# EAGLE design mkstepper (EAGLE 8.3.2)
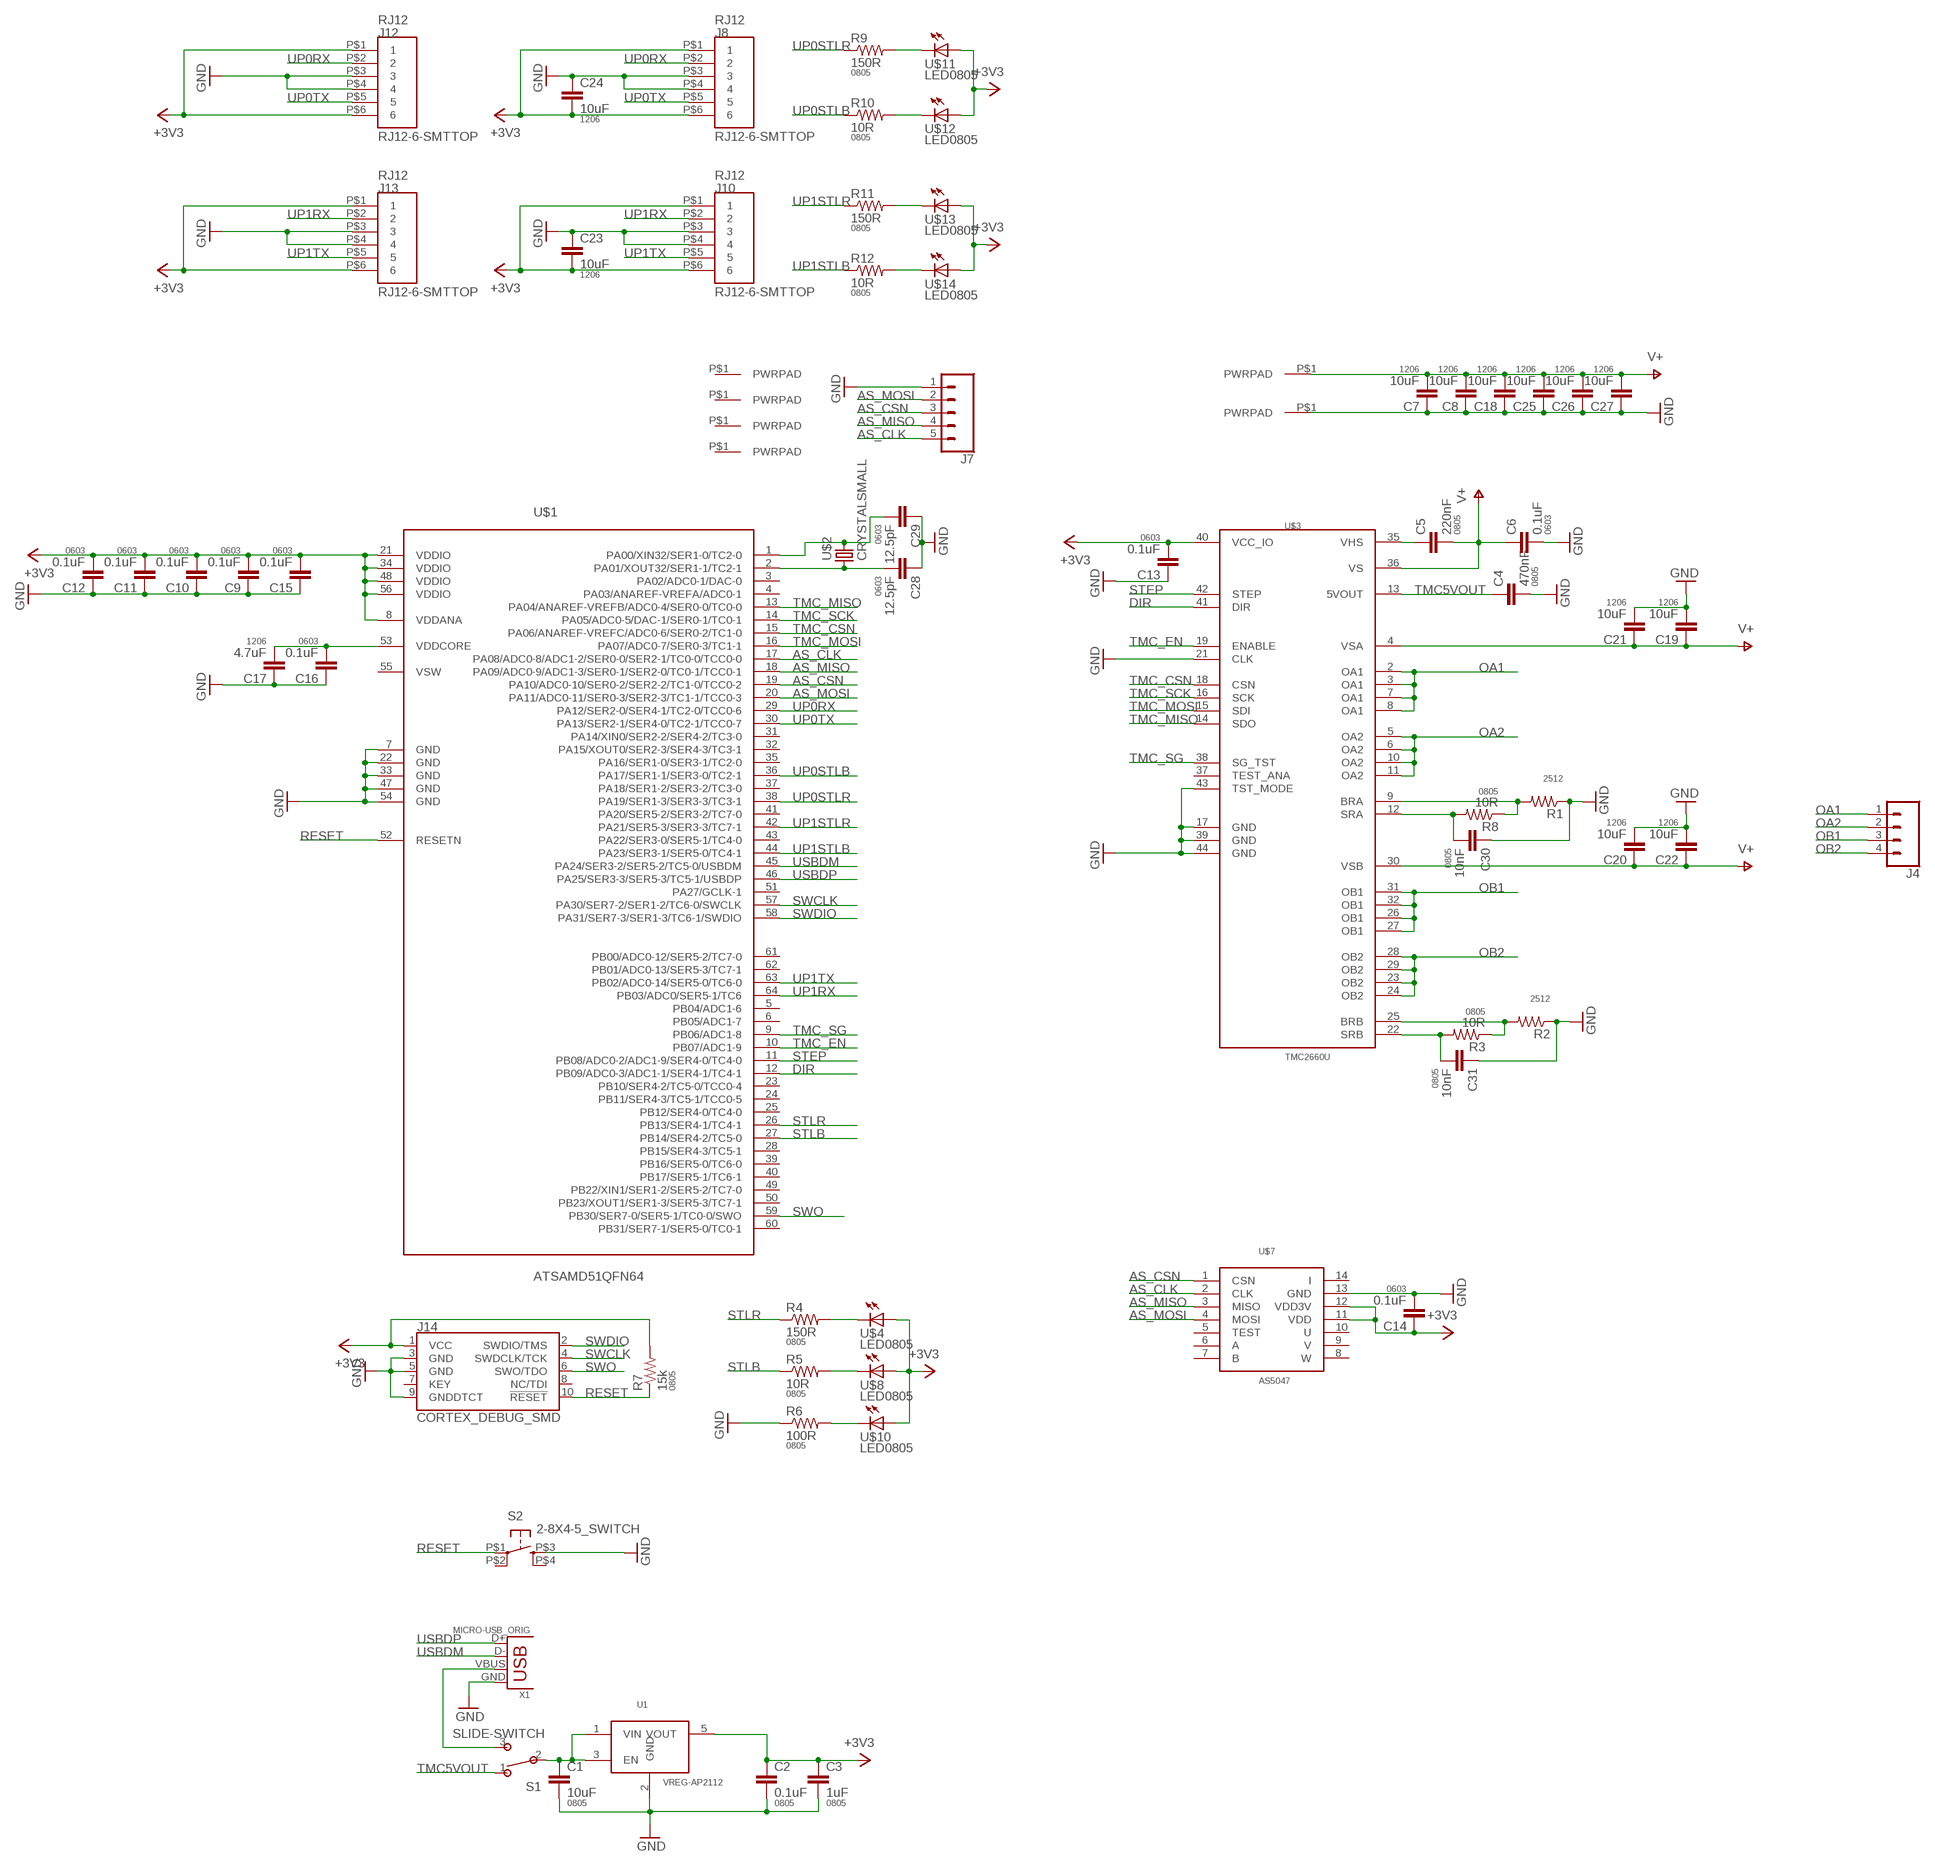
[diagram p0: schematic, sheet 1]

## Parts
C1  10uF  CAP0805  [0805]
C2  0.1uF  CAP0805  [0805]
C3  1uF  CAP0805  [0805]
C4  470nF  CAP0805  [0805]
C5  220nF  CAP0805  [0805]
C6  0.1uF  CAP0603-CAP  [0603-CAP]
C7  10uF  CAP1206  [1206]
C8  10uF  CAP1206  [1206]
C9  0.1uF  CAP0603-CAP  [0603-CAP]
C10  0.1uF  CAP0603-CAP  [0603-CAP]
C11  0.1uF  CAP0603-CAP  [0603-CAP]
C12  0.1uF  CAP0603-CAP  [0603-CAP]
C13  0.1uF  CAP0603-CAP  [0603-CAP]
C14  0.1uF  CAP0603-CAP  [0603-CAP]
C15  0.1uF  CAP0603-CAP  [0603-CAP]
C16  0.1uF  CAP0603-CAP  [0603-CAP]
C17  4.7uF  CAP1206  [1206]
C18  10uF  CAP1206  [1206]
C19  10uF  CAP1206  [1206]
C20  10uF  CAP1206  [1206]
C21  10uF  CAP1206  [1206]
C22  10uF  CAP1206  [1206]
C23  10uF  CAP1206  [1206]
C24  10uF  CAP1206  [1206]
C25  10uF  CAP1206  [1206]
C26  10uF  CAP1206  [1206]
C27  10uF  CAP1206  [1206]
C28  12.5pF  CAP0603-CAP  [0603-CAP]
C29  12.5pF  CAP0603-CAP  [0603-CAP]
C30  10nF  CAP0805  [0805]
C31  10nF  CAP0805  [0805]
J2  PWRPAD  [PWRPAD_M3-PEM-MOUNT]
J3  PWRPAD  [PWRPAD_M3-PEM-MOUNT]
J4  CONN_04LONGPADS  [1X04_LONGPADS]
J5  PWRPADM3  [PWRPAD_3-25MM]
J6  PWRPADM3  [PWRPAD_3-25MM]
J7  CONN_05NO_SILK  [1X05_NO_SILK]
J8  RJ12-6-SMTTOP  [RJ12-6-SMT-TOPENTRY]
J9  PWRPADM3  [PWRPAD_3-25MM]
J10  RJ12-6-SMTTOP  [RJ12-6-SMT-TOPENTRY]
J11  PWRPADM3  [PWRPAD_3-25MM]
J12  RJ12-6-SMTTOP  [RJ12-6-SMT-TOPENTRY]
J13  RJ12-6-SMTTOP  [RJ12-6-SMT-TOPENTRY]
J14  CORTEX_DEBUG_SMD  [SAMTECH_FTSH-105-01]
R1  RESISTOR2512  [R2512]
R2  RESISTOR2512  [R2512]
R3  10R  RESISTOR0805-RES  [0805]
R4  150R  RESISTOR0805-RES  [0805]
R5  10R  RESISTOR0805-RES  [0805]
R6  100R  RESISTOR0805-RES  [0805]
R7  15k  RESISTOR0805-RES  [0805]
R8  10R  RESISTOR0805-RES  [0805]
R9  150R  RESISTOR0805-RES  [0805]
R10  10R  RESISTOR0805-RES  [0805]
R11  150R  RESISTOR0805-RES  [0805]
R12  10R  RESISTOR0805-RES  [0805]
S1  SLIDE-SWITCH  [AYZ0102AGRLC]
S2  2-8X4-5_SWITCH  [TACT-SWITCH-KMR6]
U1  VREG-AP2112  [SOT23-5]
U$1  ATSAMD51QFN64  [QFN-64-9X9MM]
U$2  CRYSTALSMALL  [2-SMD-1-5X3-2MM]
U$3  TMC2660U  [TQFP44]
U$4  LED0805  [LED0805]
U$7  AS5047  [TSSOP14]
U$8  LED0805  [LED0805]
U$10  LED0805  [LED0805]
U$11  LED0805  [LED0805]
U$12  LED0805  [LED0805]
U$13  LED0805  [LED0805]
U$14  LED0805  [LED0805]
X1  MICRO-USB_ORIG  [DX4R005HJ5]

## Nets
+3V3: C2.1 C3.1 C9.2 C10.2 C11.2 C12.2 C13.2 C14.1 C15.2 C23.2 C24.2 J8.P$1 J8.P$6 J10.P$1 J10.P$6 J12.P$1 J12.P$6 J13.P$1 J13.P$6 J14.1(VCC) R7.2 U1.5(VOUT) U$1.8(VDDANA) U$1.21(VDDIO) U$1.34(VDDIO) U$1.48(VDDIO) U$1.56(VDDIO) U$3.40(VCC_IO) U$4.1(A) U$7.11(VDD) U$7.12(VDD3V) U$8.1(A) U$10.1(A) U$11.1(A) U$12.1(A) U$13.1(A) U$14.1(A)
AS_CLK: J7.5 U$1.17(PA08/ADC0-8/ADC1-2/SER0-0/SER2-1/TC0-0/TCC0-0) U$7.2(CLK)
AS_CSN: J7.3 U$1.19(PA10/ADC0-10/SER0-2/SER2-2/TC1-0/TCC0-2) U$7.1(CSN)
AS_MISO: J7.4 U$1.18(PA09/ADC0-9/ADC1-3/SER0-1/SER2-0/TC0-1/TCC0-1) U$7.3(MISO)
AS_MOSI: J7.2 U$1.20(PA11/ADC0-11/SER0-3/SER2-3/TC1-1/TCC0-3) U$7.4(MOSI)
BRA: R1.2 R8.1 U$3.9(BRA)
BRB: R2.2 R3.1 U$3.25(BRB)
DIR: U$1.12(PB09/ADC0-3/ADC1-1/SER4-1/TC4-1) U$3.41(DIR)
GND: C1.2 C2.2 C3.2 C4.2 C6.2 C7.1 C8.1 C9.1 C10.1 C11.1 C12.1 C13.1 C14.2 C15.1 C16.1 C17.1 C18.1 C19.2 C20.2 C21.2 C22.2 C23.1 C24.1 C25.1 C26.1 C27.1 C28.1 C29.1 C30.1 C31.1 J3.P$1(PWRPAD) J7.1 J8.P$3 J8.P$4 J10.P$3 J10.P$4 J12.P$3 J12.P$4 J13.P$3 J13.P$4 J14.3(GND) J14.5(GND) J14.9(GNDDTCT) R1.1 R2.1 R6.1 S2.P$3(S) U1.2(GND) U$1.7(GND) U$1.22(GND) U$1.33(GND) U$1.47(GND) U$1.54(GND) U$3.17(GND) U$3.21(CLK) U$3.39(GND) U$3.43(TST_MODE) U$3.44(GND) U$7.13(GND) X1.GND
N$1: R6.2 U$10.2(C)
N$2: C5.1 U$3.35(VHS)
N$3: C1.1 S1.2 U1.1(VIN) U1.3(EN)
N$4: S1.3 X1.VBUS
N$5: R5.2 U$8.2(C)
N$6: R4.2 U$4.2(C)
N$7: C16.2 C17.2 U$1.53(VDDCORE)
N$8: C28.2 U$1.2(PA01/XOUT32/SER1-1/TC2-1) U$2.P$1
N$10: R9.2 U$11.2(C)
N$11: R10.2 U$12.2(C)
N$12: C29.2 U$1.1(PA00/XIN32/SER1-0/TC2-0) U$2.P$2
N$13: R11.2 U$13.2(C)
N$14: R12.2 U$14.2(C)
OA1: J4.1 U$3.2(OA1) U$3.3(OA1) U$3.7(OA1) U$3.8(OA1)
OA2: J4.2 U$3.5(OA2) U$3.6(OA2) U$3.10(OA2) U$3.11(OA2)
OB1: J4.3 U$3.26(OB1) U$3.27(OB1) U$3.31(OB1) U$3.32(OB1)
OB2: J4.4 U$3.23(OB2) U$3.24(OB2) U$3.28(OB2) U$3.29(OB2)
RESET: J14.10(!RESET) R7.1 S2.P$1(P) U$1.52(RESETN)
SRA: C30.2 R8.2 U$3.12(SRA)
SRB: C31.2 R3.2 U$3.22(SRB)
STEP: U$1.11(PB08/ADC0-2/ADC1-9/SER4-0/TC4-0) U$3.42(STEP)
STLB: R5.1 U$1.27(PB14/SER4-2/TC5-0)
STLR: R4.1 U$1.26(PB13/SER4-1/TC4-1)
SWCLK: J14.4(SWDCLK/TCK) U$1.57(PA30/SER7-2/SER1-2/TC6-0/SWCLK)
SWDIO: J14.2(SWDIO/TMS) U$1.58(PA31/SER7-3/SER1-3/TC6-1/SWDIO)
SWO: J14.6(SWO/TDO) U$1.59(PB30/SER7-0/SER5-1/TC0-0/SWO)
TMC5VOUT: C4.1 S1.1 U$3.13(5VOUT)
TMC_CSN: U$1.15(PA06/ANAREF-VREFC/ADC0-6/SER0-2/TC1-0) U$3.18(CSN)
TMC_EN: U$1.10(PB07/ADC1-9) U$3.19(ENABLE)
TMC_MISO: U$1.13(PA04/ANAREF-VREFB/ADC0-4/SER0-0/TC0-0) U$3.14(SDO)
TMC_MOSI: U$1.16(PA07/ADC0-7/SER0-3/TC1-1) U$3.15(SDI)
TMC_SCK: U$1.14(PA05/ADC0-5/DAC-1/SER0-1/TC0-1) U$3.16(SCK)
TMC_SG: U$1.9(PB06/ADC1-8) U$3.38(SG_TST)
UP0RX: J8.P$2 J12.P$2 U$1.29(PA12/SER2-0/SER4-1/TC2-0/TCC0-6)
UP0STLB: R10.1 U$1.36(PA17/SER1-1/SER3-0/TC2-1)
UP0STLR: R9.1 U$1.38(PA19/SER1-3/SER3-3/TC3-1)
UP0TX: J8.P$5 J12.P$5 U$1.30(PA13/SER2-1/SER4-0/TC2-1/TCC0-7)
UP1RX: J10.P$2 J13.P$2 U$1.64(PB03/ADC0/SER5-1/TC6)
UP1STLB: R12.1 U$1.44(PA23/SER3-1/SER5-0/TC4-1)
UP1STLR: R11.1 U$1.42(PA21/SER5-3/SER3-3/TC7-1)
UP1TX: J10.P$5 J13.P$5 U$1.63(PB02/ADC0-14/SER5-0/TC6-0)
USBDM: U$1.45(PA24/SER3-2/SER5-2/TC5-0/USBDM) X1.D-
USBDP: U$1.46(PA25/SER3-3/SER5-3/TC5-1/USBDP) X1.D+
V+: C5.2 C6.1 C7.2 C8.2 C18.2 C19.1 C20.1 C21.1 C22.1 C25.2 C26.2 C27.2 J2.P$1(PWRPAD) U$3.4(VSA) U$3.30(VSB) U$3.36(VS)
Unconnected: J5.P$1(PWRPAD) J6.P$1(PWRPAD) J9.P$1(PWRPAD) J11.P$1(PWRPAD) J14.7(KEY) J14.8(NC/TDI) S2.P$2(P1) S2.P$4(S1) U$1.3(PA02/ADC0-1/DAC-0) U$1.4(PA03/ANAREF-VREFA/ADC0-1) U$1.5(PB04/ADC1-6) U$1.6(PB05/ADC1-7) U$1.23(PB10/SER4-2/TC5-0/TCC0-4) U$1.24(PB11/SER4-3/TC5-1/TCC0-5) U$1.25(PB12/SER4-0/TC4-0) U$1.28(PB15/SER4-3/TC5-1) U$1.31(PA14/XIN0/SER2-2/SER4-2/TC3-0) U$1.32(PA15/XOUT0/SER2-3/SER4-3/TC3-1) U$1.35(PA16/SER1-0/SER3-1/TC2-0) U$1.37(PA18/SER1-2/SER3-2/TC3-0) U$1.39(PB16/SER5-0/TC6-0) U$1.40(PB17/SER5-1/TC6-1) U$1.41(PA20/SER5-2/SER3-2/TC7-0) U$1.43(PA22/SER3-0/SER5-1/TC4-0) U$1.49(PB22/XIN1/SER1-2/SER5-2/TC7-0) U$1.50(PB23/XOUT1/SER1-3/SER5-3/TC7-1) U$1.51(PA27/GCLK-1) U$1.55(VSW) U$1.60(PB31/SER7-1/SER5-0/TC0-1) U$1.61(PB00/ADC0-12/SER5-2/TC7-0) U$1.62(PB01/ADC0-13/SER5-3/TC7-1) U$3.37(TEST_ANA) U$7.5(TEST) U$7.6(A) U$7.7(B) U$7.8(W) U$7.9(V) U$7.10(U) U$7.14(I)

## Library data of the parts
C1-C5 C30 C31 = borkedlabs-passives:CAP: Capacitor; PACKAGE: 0805
C6 C9-C16 C28 C29 = borkedlabs-passives:CAP: Capacitor; PACKAGE: 0603
C7 C8 C17-C27 = borkedlabs-passives:CAP: Capacitor; PACKAGE: 1206
J2 J3 J5 J6 J9 J11 = power:PWRPAD
J4 = SparkFun-Connectors:CONN_04: Multi connection point. Often used as Generic Header-pin footprint for 0.1 inch spaced/style header connections On any of the 0.1 inch spaced packages, you can populate with these: Break Away Headers - Straight (PRT-00116) Break Away Male Headers - Right Angle (PRT-00553) Female Headers (PRT-00115)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; PROD_ID: CONN-09696
J7 = SparkFun-Connectors:CONN_05: Multi connection point. Often used as Generic Header-pin footprint for 0.1 inch spaced/style header connections On any of the 0.1 inch spaced packages, you can populate with these: Break Away Headers - Straight (PRT-00116) Break Away Male Headers - Right Angle (PRT-00553) Female Headers (PRT-00115)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
J8 J10 J12 J13 = connector:RJ12-6-SMT
J14 = SparkFun-Connectors:CORTEX_DEBUG: Cortex Debug Connector - 10 pin Supports JTAG debug, Serial Wire debug, and Serial Wire Viewer. PTH and SMD connector options available. General Connector Information Products: PTH Connector -via Digi-Key SparkFun PSoc SparkFun T
R1 R2 = borkedlabs-passives:RESISTOR: Resistor; PACKAGE: 2512
R3-R12 = borkedlabs-passives:RESISTOR: Resistor; PACKAGE: 0805
S1 = fab:SLIDE-SWITCH: SMD slide-switch AYZ0102AGRLC as found in the fablab inventory. Includes the mounting holes. Made by Zaerc.
S2 = fab:2-8X4-5_SWITCH
U1 = power:VREG-AP2112
U$1 = atsam:ATSAMD51
U$2 = fab:CRYSTAL
U$3 = power:TMC2660
U$4 U$8 U$10-U$14 = lights:LED: LED
U$7 = sensor:AS5047
X1 = fab:MICRO-USB: SMD micro USB connector as found in the fablab inventory. Three footprint variants included: original, as described by manufacturer's datasheet for milling with the 1/100" bit for milling with the 1/64" bit Made by Zaerc.

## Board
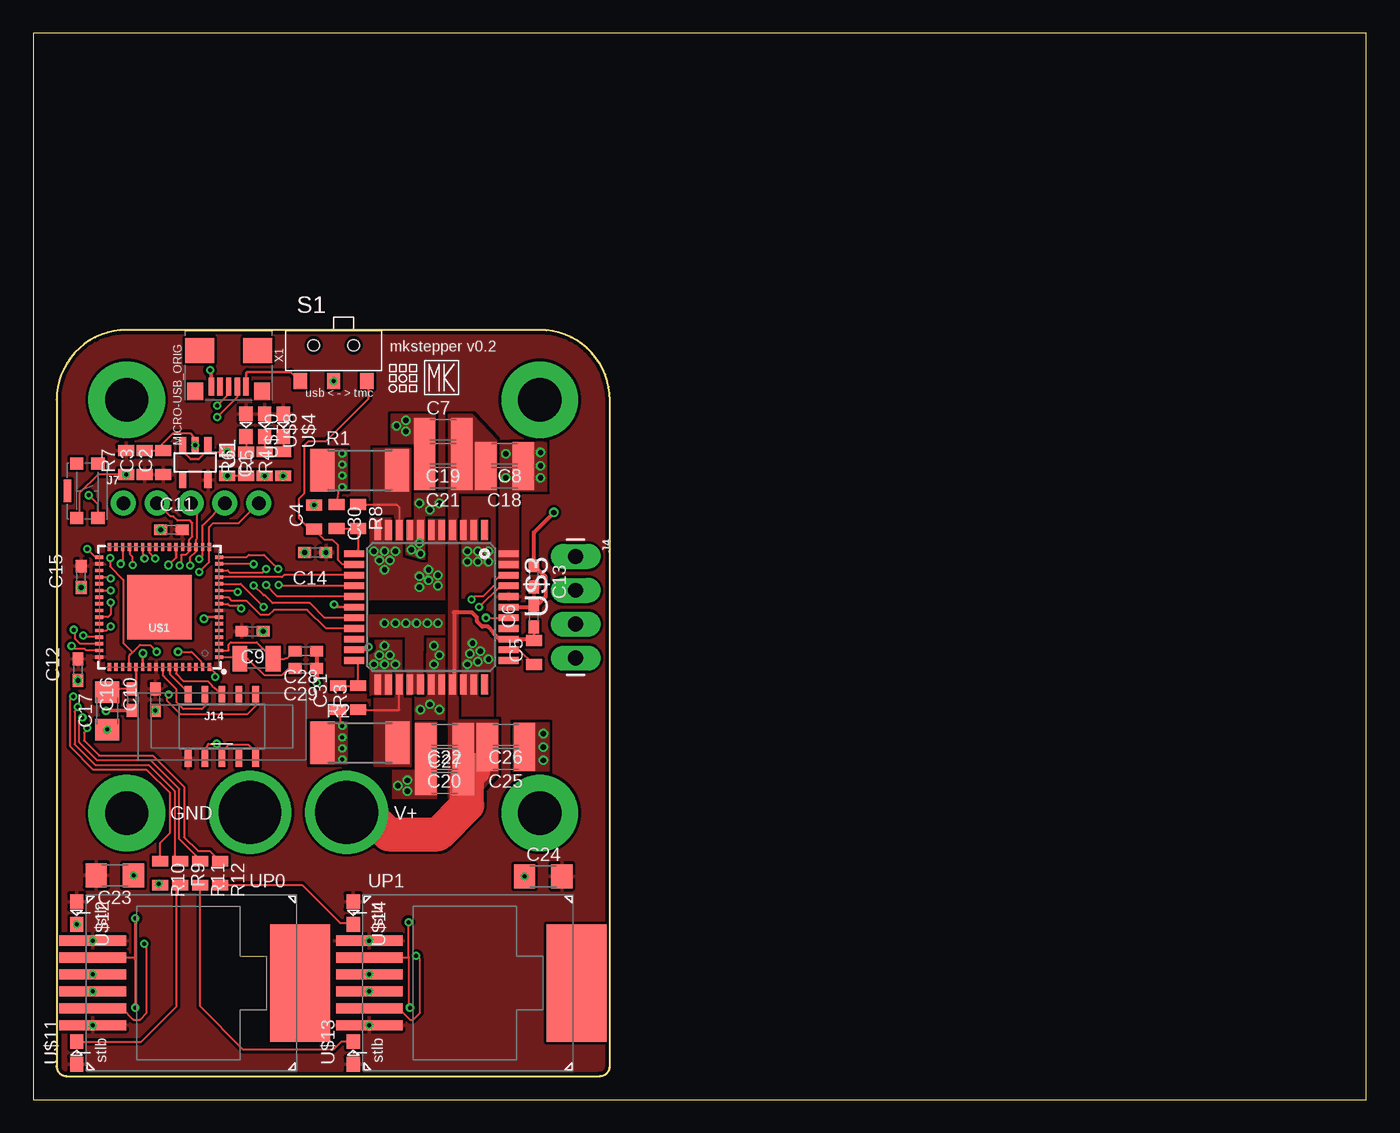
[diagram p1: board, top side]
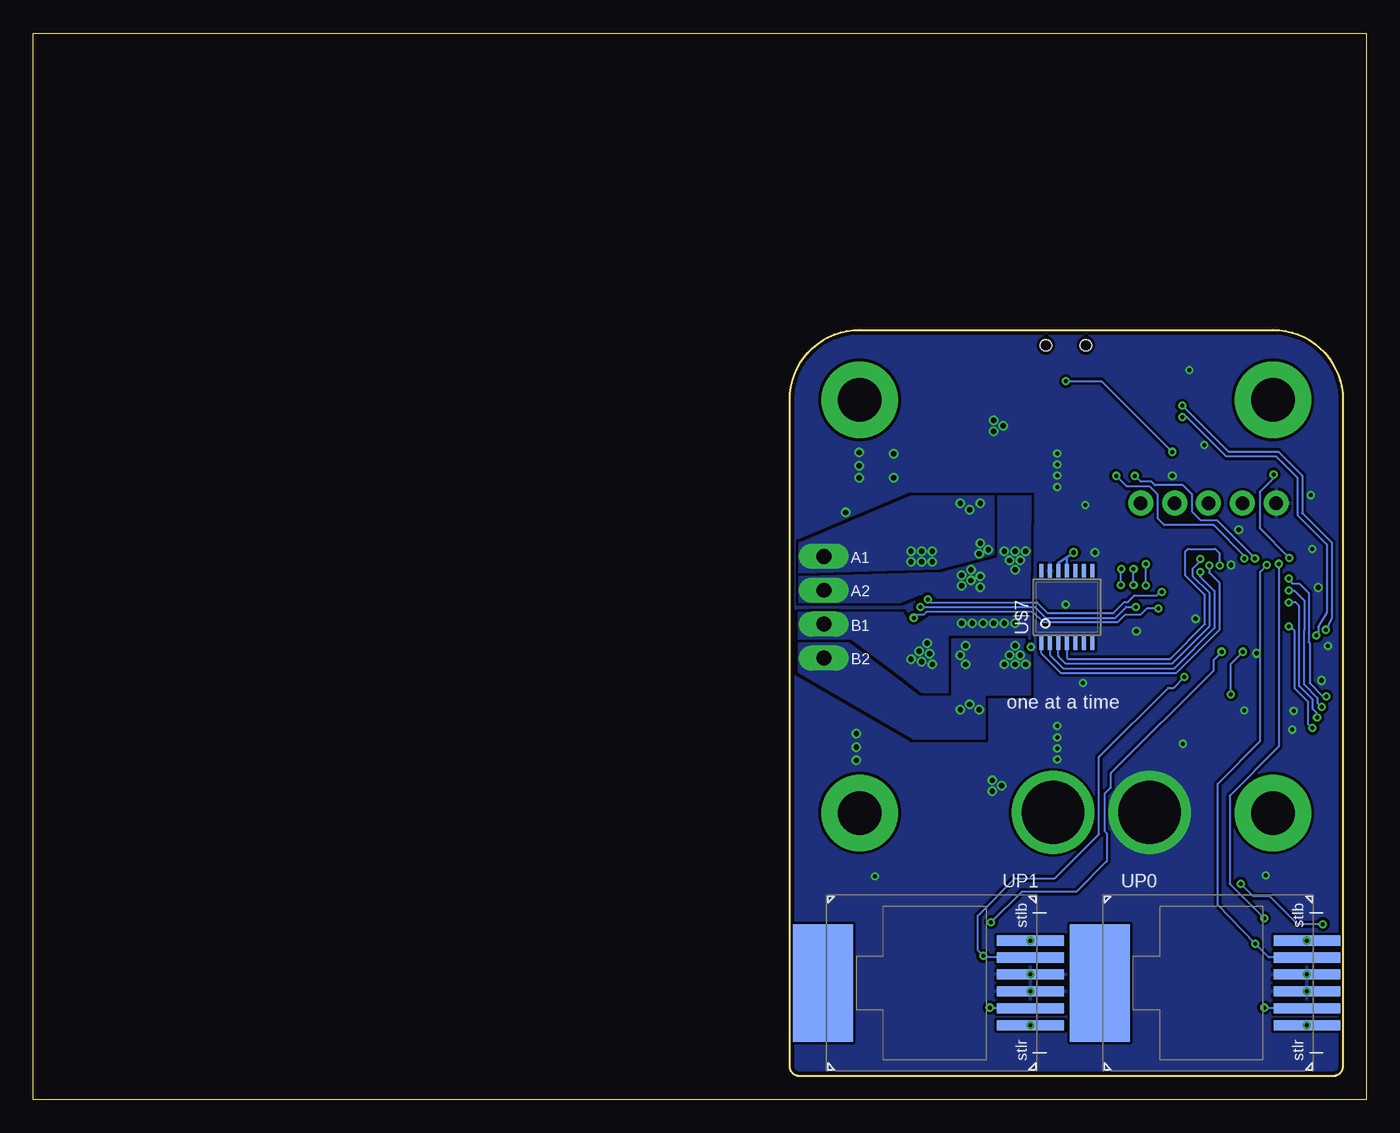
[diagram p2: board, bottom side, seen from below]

Size 100 x 80 mm. Coordinates in mm from the lower left corner, seen from the top.
Outline: 0,0 100,0 100,80 0,80 0,0
Outline: 1.75,52.5 1.75,2.5 arc90 2.5,1.75 42.5,1.75 arc90 43.25,2.5 43.25,52.5 arc90 38,57.75 7,57.75 arc90 1.75,52.5
Copper layers (1*16): Top 0.035mm / dielectric 1.5mm / Bottom 0.035mm
Design rules "default *": minimum track width 6mil, minimum drill 0.3mm, track to track 8mil, track to pad 8mil, pad to pad 8mil, via to via 8mil, smd to smd 8mil, copper to edge 10mil, drill to drill 10mil, minimum pad ring 6mil, minimum via ring 6mil, stop-mask expansion 4mil, vias tented up to drill 27mil, thermal gap 9mil

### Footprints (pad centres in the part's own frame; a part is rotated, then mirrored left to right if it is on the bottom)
0805 = smd 0.8 x 1.2: 1 -0.9,0; 2 0.9,0
0603-CAP = smd 0.96 x 0.8: 1 -0.8,0; 2 0.8,0
1206 = smd 1.6 x 1.8: 1 -1.4,0; 2 1.4,0
PWRPAD_M3-PEM-MOUNT = drill 4.7 pad 6.2: P$1 0,0
1X04_LONGPADS = drill 1.118 pad 1.88 long: 1 0,0; 2 2.54,0; 3 5.08,0; 4 7.62,0
PWRPAD_3-25MM = drill 3.25 pad 5.75: P$1 0,0
1X05_NO_SILK = drill 1.016 pad 1.88: 1 0,0; 2 2.54,0; 3 5.08,0; 4 7.62,0; 5 10.16,0
RJ12-6-SMT-TOPENTRY = smd 0.76 x 5: P$1 -3.175,15.3; P$2 -1.905,15.3; P$3 -0.635,15.3; P$4 0.635,15.3; P$5 1.905,15.3; P$6 3.175,15.3 | smd 8.8 x 4.5: P$7 0,-0.25
SAMTECH_FTSH-105-01 = smd 0.508 x 1.27: 1 -2.54,-2.413; 2 -2.54,2.413; 3 -1.27,-2.413; 4 -1.27,2.413; 5 0,-2.413; 6 0,2.413; 7 1.27,-2.413; 8 1.27,2.413; 9 2.54,-2.413; 10 2.54,2.413
R2512 = smd 1.8 x 3.2: 1 -2.8,0; 2 2.8,0
AYZ0102AGRLC = smd 1 x 1.2: 1 2.5,-2.3; 2 0,-2.3; 3 -2.5,-2.3 | hole 0.85: -1.5,0.4; 1.5,0.4
TACT-SWITCH-KMR6 = smd 0.9 x 1: P$1 -2.05,0.8; P$2 2.05,0.8; P$3 -2.05,-0.8; P$4 2.05,-0.8 | smd 1.7 x 0.55: P$5 0,1.5
SOT23-5 = smd 0.533 x 1.194: 1 -0.95,-1.306; 2 0,-1.306; 3 0.95,-1.306; 4 0.95,1.306; 5 -0.95,1.306
QFN-64-9X9MM = smd 0.6 x 0.25: 1 -4.5,3.75; 2 -4.5,3.25; 3 -4.5,2.75; 4 -4.5,2.25; 5 -4.5,1.75; 6 -4.5,1.25; 7 -4.5,0.75; 8 -4.5,0.25; 9 -4.5,-0.25; 10 -4.5,-0.75; 11 -4.5,-1.25; 12 -4.5,-1.75; 13 -4.5,-2.25; 14 -4.5,-2.75; 15 -4.5,-3.25; 16 -4.5,-3.75; 33 4.5,-3.75; 34 4.5,-3.25; 35 4.5,-2.75; 36 4.5,-2.25; 37 4.5,-1.75; 38 4.5,-1.25; 39 4.5,-0.75; 40 4.5,-0.25; 41 4.5,0.25; 42 4.5,0.75; 43 4.5,1.25; 44 4.5,1.75; 45 4.5,2.25; 46 4.5,2.75; 47 4.5,3.25; 48 4.5,3.75 | smd 0.25 x 0.6: 17 -3.75,-4.5; 18 -3.25,-4.5; 19 -2.75,-4.5; 20 -2.25,-4.5; 21 -1.75,-4.5; 22 -1.25,-4.5; 23 -0.75,-4.5; 24 -0.25,-4.5; 25 0.25,-4.5; 26 0.75,-4.5; 27 1.25,-4.5; 28 1.75,-4.5; 29 2.25,-4.5; 30 2.75,-4.5; 31 3.25,-4.5; 32 3.75,-4.5; 49 3.75,4.5; 50 3.25,4.5; 51 2.75,4.5; 52 2.25,4.5; 53 1.75,4.5; 54 1.25,4.5; 55 0.75,4.5; 56 0.25,4.5; 57 -0.25,4.5; 58 -0.75,4.5; 59 -1.25,4.5; 60 -1.75,4.5; 61 -2.25,4.5; 62 -2.75,4.5; 63 -3.25,4.5; 64 -3.75,4.5 | smd 4.826 x 4.826: P$1 0,0
2-SMD-1-5X3-2MM = smd 1.1 x 1.9: P$1 -1.25,0; P$2 1.25,0
TQFP44 = smd 1.5 x 0.5: 1 -5.8,4; 2 -5.8,3.2; 3 -5.8,2.4; 4 -5.8,1.6; 5 -5.8,0.8; 6 -5.8,0; 7 -5.8,-0.8; 8 -5.8,-1.6; 9 -5.8,-2.4; 10 -5.8,-3.2; 11 -5.8,-4; 23 5.8,-4; 24 5.8,-3.2; 25 5.8,-2.4; 26 5.8,-1.6; 27 5.8,-0.8; 28 5.8,0; 29 5.8,0.8; 30 5.8,1.6; 31 5.8,2.4; 32 5.8,3.2; 33 5.8,4 | smd 0.5 x 1.5: 12 -4,-5.8; 13 -3.2,-5.8; 14 -2.4,-5.8; 15 -1.6,-5.8; 16 -0.8,-5.8; 17 0,-5.8; 18 0.8,-5.8; 19 1.6,-5.8; 20 2.4,-5.8; 21 3.2,-5.8; 22 4,-5.8; 34 4,5.8; 35 3.2,5.8; 36 2.4,5.8; 37 1.6,5.8; 38 0.8,5.8; 39 0,5.8; 40 -0.8,5.8; 41 -1.6,5.8; 42 -2.4,5.8; 43 -3.2,5.8; 44 -4,5.8
LED0805 = smd 1.1 x 1: 1 -0.85,0; 2 0.85,0
TSSOP14 = smd 0.305 x 0.991: 1 -1.905,-2.718; 2 -1.27,-2.718; 3 -0.635,-2.718; 4 0,-2.718; 5 0.635,-2.718; 6 1.27,-2.718; 7 1.905,-2.718; 8 1.905,2.718; 9 1.27,2.718; 10 0.635,2.718; 11 0,2.718; 12 -0.635,2.718; 13 -1.27,2.718; 14 -1.905,2.718
DX4R005HJ5 = smd 0.4 x 1.35: D+ 0,1.6; D- -0.65,1.6; GND 1.3,1.6; ID 0.65,1.6; VBUS -1.3,1.6 | smd 1.2 x 1.3: GND@1 -2.5,1.95; GND@2 2.5,1.95 | smd 2.15 x 1.9: GND@3 -2.175,-1.1; GND@4 2.175,-1.1

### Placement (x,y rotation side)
C1  14.55,47.7 270 top
C2  9.75,47.8 90 top
C3  8.35,47.8 90 top
C4  21.06,43.71 90 top
C5  37.55,33.55 90 top
C6  37.55,36.25 90 top
C7  30.75,50.25 0 top
C8  35.35,48.45 180 top
C9  16.45,35.13 180 top
C10  9.15,30 90 top
C11  10.36,42.75 0 top
C12  3.35,32.25 90 top
C13  37.55,39.25 270 top
C14  21.15,41.05 180 top
C15  3.59,39.22 90 top
C16  7.4,30 90 top
C17  5.55,29.15 90 top
C18  35.35,46.65 180 top
C19  30.75,48.45 180 top
C20  30.85,25.55 180 top
C21  30.75,46.65 180 top
C22  30.85,27.35 180 top
C23  6.12,16.82 180 top
C24  38.25,16.75 0 top
C25  35.45,25.55 180 top
C26  35.45,27.35 180 top
C27  30.85,23.75 0 top
C28  20.45,33.65 180 top
C29  20.45,32.35 180 top
C30  22.75,43.75 270 top
C31  22.85,30.15 90 top
J2  23.5,21.54 0 top
J3  16.25,21.54 0 top
J4  40.7,40.75 270 top
J5  38,52.5 0 top
J6  7,52.5 0 top
J7  6.75,44.75 0 top
J8  19.75,8.75 270 bottom
J9  7,21.5 0 top
J10  40.5,8.75 270 bottom
J11  38,21.5 0 top
J12  19.75,8.75 90 top
J13  40.5,8.75 90 top
J14  14.15,28 0 top
R1  24.51,47.22 0 top
R2  24.52,26.76 0 top
R3  24.35,30.15 90 top
R4  18.75,47.7 90 top
R5  17.35,47.7 90 top
R6  15.95,47.7 90 top
R7  6.95,47.8 90 top
R8  24.35,43.75 270 top
R9  11,17 270 top
R10  9.5,17 270 top
R11  12.5,17 270 top
R12  14,17 270 top
S1  22.53,56.19 0 top
S2  4.06,45.67 90 top
U1  12.15,47.8 180 top
U$1  9.45,36.95 180 top
U$2  16.74,33.07 180 top
U$3  29.85,36.95 270 top
U$4  18.75,50.6 270 top
U$5  [CBA-SILK-LOGO]  27.73,54.12 90 top
U$7  22.45,36.95 0 bottom
U$8  17.35,50.6 270 top
U$9  [MK-LOGO-SILK]  30.63,54.16 0 top
U$10  15.95,50.6 270 top
U$11  3.25,3.5 90 top
U$12  3.25,14 270 top
U$13  24,3.5 90 top
U$14  24,14 270 top
X1  14.65,55.1 180 top

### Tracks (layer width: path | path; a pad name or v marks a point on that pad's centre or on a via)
+3V3  (via drill 0.3, 0.35)
  Bottom 0.2: C14.1 22.15,40.9 22.38,40.74 | U$7.12 23.09,40.27 22.38,40.74 | U$7.11 22.45,40.67 22.38,40.74
  other vias: 21.95,41.05 4.45,11.93 4.45,5.58 25.2,5.58 25.2,11.93
  pour Top (rank 6): 1.75,58 1.75,1.75 43.25,1.75 43.25,58
AS_CLK  (via drill 0.3)
  Top 0.152: v12.44,39.58 13.2,40.33 U$1.17 13.2,42.95 13.5,43.25 15.41,43.25 J7.5
  Bottom 0.152: U$7.2 23.7,34.21 23.7,33.32 22.74,32.36 14.41,32.36 11.39,35.38 11.39,38.16 12.44,39.21 v12.44,39.58
AS_CSN  (via drill 0.3 pad 0.42)
  Top 0.152: v11.78,40.05 11.74,40.1 11.74,40.66 12.2,41.13 U$1.19 12.2,42.01 12.28,42.09 12.28,44.3 J7.3
  Bottom 0.152: U$7.1 24.39,34.2 24.39,33.48 22.91,32 14.26,32 11.04,35.23 11.04,38.8 11.78,39.54 v11.78,40.05
AS_MISO  (via drill 0.3)
  Top 0.152: v12.44,40.54 12.7,40.8 U$1.18 12.7,43.08 J7.4
  Bottom 0.152: U$7.3 23.09,33.25 22.56,32.71 14.56,32.71 11.75,35.52 11.75,38.01 13.03,39.29 13.03,39.82 12.44,40.41 v12.44,40.54
AS_MOSI  (via drill 0.3 pad 0.42)
  Top 0.152: v10.97,40.08 11.08,40.19 11.08,40.82 11.13,40.87 11.44,40.87 11.7,41.13 U$1.20 11.7,42.02 11.92,42.24 11.92,43.27 11.76,43.43 10.82,43.43 10.5,43.75 10.29,43.75 J7.2
  Bottom 0.152: U$7.4 22.45,33.12 22.41,33.07 14.7,33.07 12.1,35.67 12.1,37.87 13.56,39.33 13.56,41.12 13.36,41.33 11.33,41.33 10.97,40.96 v10.97,40.08
BRA
  Top 0.152: R8.1 27.25,44.65 27.45,44.45 U$3.9
  pour Top (no thermals): 27.15,41.95 27.15,43.95 25.55,43.95 25.55,48.85 28.25,48.85 28.25,43.75 27.75,43.75 27.75,41.95
BRB
  Top 0.152: R3.1 27.45,29.25 U$3.25
  pour Top (no thermals): 27.15,31.95 27.15,30.05 25.55,30.05 25.55,25.05 28.35,25.05 28.35,30.05 27.75,30.05 27.75,31.95
DIR  (via drill 0.3, 0.3 pad 0.42)
  Top 0.152: U$1.12 15.56,38.7 v17.29,36.97 | U$3.41 35.05,38.55 v33.45,36.95
  Top 0.2: 35.02,38.55 U$3.41
  Bottom 0.152: v33.45,36.95 24.85,36.95 24.05,36.15 18.82,36.15 18,36.97 v17.29,36.97 | v17.29,36.97
GND  (via drill 0.3, 0.3 pad 0.42, 0.35, 0.4 pad 0.42)
  Top 0.152: v23.19,28.02 23.25,28.08 23.05,28.28 C31.1 | 23.25,45.91 v23.19,45.97 22.95,45.73 C30.1 | S2.P$3 4.86,44.64 v4.16,45.34 | C3.2 C2.2 9.68,49.18 10.5,50 11.75,50 12,49.75 12,49.17 U1.2 | R6.1 C1.2 | U$1.33 4.65,40.7 v4.05,41.3 | J14.9 16.69,26.06 16.15,26.6 14.65,26.6 14.25,26.2 14.25,26.1 | 14.25,26.1 14.25,25.59 J14.5 | J14.3 12.88,26.23 13.15,26.7 v13.75,26.7 14.25,26.1 | U$1.47 3.98,33.7 3.87,33.81 3.09,33.81 v2.86,34.04
  Top 0.2: U$3.17 22.75,36.95 v22.55,37.15 | U$3.21 24.96,33.75 v25.16,33.94 | 37.5,40.15 C13.1 | 37.45,37.05 C6.2
  Top 0.203: 7.34,29.09 C16.1 | U$1.54 8.2,33.44 v8.23,33.48 | U$1.7 12.94,36.2 v12.8,36.07 | U$1.22 10.7,40.67 v10.14,40.11
  Top 0.254: X1.GND 13.35,54.88 v13.26,54.72
  Top 0.305: C28.1 C29.1 21.3,31.3 v21.25,31.25 | C6.2 37.85,37.15 38.41,37.7 38.41,37.71 38.45,37.75 38.45,39.2 C13.1 37.55,42.55 v39.05,44.05 | U$3.39 37.35,36.95 37.45,37.05 | C16.1 v5.45,29.15
  Top 1.27: C22.2 C20.2 C27.1 | C18.1 C8.1 | C25.1 C26.1
  other vias: 20.35,41.05 23.19,48.48 23.19,46.81 23.19,47.65 23.19,25.5 23.19,26.34 23.19,27.18 5.55,27.75 3.59,38.42 9.56,42.75 17.25,35.13 14.55,46.8 3.35,31.45 12.15,49.11 21.06,44.61 38.25,27.45 38.25,26.45 38.25,25.45 28.05,23.95 28.05,23.15 27.35,23.55 38.05,48.55 38.05,47.55 38.05,46.65 27.95,50.95 27.95,50.15 27.25,50.55 35.45,46.65 35.45,48.45 9.15,29.2 4.45,9.38 4.45,8.12 25.2,9.38 25.2,8.12 7.52,16.82 36.85,16.75
  pour Top (no thermals): 20.82,48.79 23.49,48.79 23.49,45.66 20.82,45.66
  pour Top (no thermals): 20.82,28.32 23.49,28.32 23.49,25.2 20.82,25.2
  pour Top (no thermals): 36.05,28.25 38.65,28.25 38.65,24.65 36.05,24.65
  pour Top (rank 3, no thermals): 30.25,22.65 30.25,28.25 28.65,28.25 28.65,24.65 26.95,24.65 26.95,22.65
  pour Top (no thermals): 35.95,49.25 35.95,45.75 38.45,45.75 38.45,49.25
  pour Top (rank 3, no thermals): 28.55,45.75 30.15,45.75 30.15,51.35 26.85,51.35 26.85,49.25 28.55,49.25
  pour Top (rank 3, no thermals): 34.95,39.85 34.95,49.25 38.45,49.25 38.45,45.65 36.35,45.65 36.35,39.85
  pour Bottom (rank 5): 1.75,57.75 1.75,1.75 43.25,1.75 43.25,57.75
N$1
  Top 0.152: U$10.2 R6.2
N$2
  Top 0.2: U$3.35 36.45,33.75 C5.1
N$3  (via drill 0.3 pad 0.42)
  Top 0.2: U1.3 11.15,48.7 11.8,48.05 12.4,48.05 13.05,48.7 13.05,48.75 | 13.05,48.75 U1.1 | C1.1 13.25,48.54 13.05,48.75
  Bottom 0.152: S1.2 19.86,53.89 C1.1
  other vias: 14.55,48.6 22.53,53.89
N$4
  Top 0.2: X1.VBUS 15.95,54.5 16.05,54.6 19.32,54.6 S1.3
N$5
  Top 0.152: U$8.2 R5.2
N$6
  Top 0.152: U$4.2 R4.2
N$7
  Top 0.203: U$1.53 7.7,31.15 C16.2 5.85,30.85 C17.2
N$8
  Top 0.152: U$1.2 14.66,33.7 14.66,34.14 14.82,34.3 16.76,34.3 U$2.P$1 18.88,33.07 18.93,33.13 19.08,33.13 C28.2
N$10
  Top 0.152: U$11.2 8.1,4.35 10.75,7 10.75,15.85 R9.2
N$11  (via drill 0.3)
  Top 0.152: v9.41,16.19 R10.2
  Bottom 0.152: U$12.2 5.15,13.15 7.25,15.25 8.48,15.25 v9.41,16.19
  other vias: 3.25,13.15
N$12
  Top 0.152: U$1.1 15.16,33.2 U$2.P$2 16.09,33.07 17.32,31.84 18.65,31.84 19.16,32.35 C29.2
N$13
  Top 0.152: U$13.2 23.1,4.35 22.5,3.75 15.75,3.75 12.5,7 R11.2
N$14
  Top 0.152: R12.2 20.15,16.1 23,13.25 23.9,13.25 U$14.2
OA1  (via drill 0.4 pad 0.42)
  other vias: 28.95,41.75 29.05,40.95 28.35,41.25 32.55,40.35 33.35,40.35 34.15,40.35 28.95,44.75 30.45,44.75 29.75,44.25 32.55,41.15 33.35,41.15 34.15,41.15
  pour Bottom (rank 2, no thermals): 42.55,39.55 32.05,39.85 27.95,40.95 27.95,45.25 34.15,45.25 42.45,41.75 42.55,41.75
  pour Top (rank 2, no thermals): 28.45,45.45 28.45,43.65 27.95,43.65 27.95,40.95 29.35,40.55 29.35,43.85 31.05,43.85 31.05,45.45
  pour Top (rank 2, no thermals): 31.85,45.45 31.85,39.95 31.95,37.65 34.65,37.75 34.65,45.45
OA2  (via drill 0.4 pad 0.42)
  other vias: 26.75,40.45 26.35,41.15 27.15,41.15 25.95,40.45 25.55,41.15 26.35,39.75 29.65,39.75 29.65,38.95 30.35,39.35 30.35,38.55 28.95,39.25 28.95,38.45
  pour Bottom (rank 3, no thermals): 42.55,37.35 34.95,37.35 33.45,37.95 32.55,37.95 32.05,37.55 25.25,37.55 25.15,45.25 27.65,45.25 27.75,40.75 32.15,39.65 42.55,39.25
  pour Top (rank 3, no thermals): 27.05,43.65 25.25,43.65 25.25,37.55 32.05,37.55 32.55,37.95 33.65,37.95 34.45,38.75 34.45,39.55 32.55,39.55 31.75,39.75 31.75,41.85 31.05,41.85 31.05,43.55 29.55,43.55 29.55,40.35 27.75,40.85 27.75,41.85 27.05,41.85
OB1  (via drill 0.4 pad 0.42)
  other vias: 27.95,35.75 27.15,35.75 26.35,35.75 28.75,35.75 29.55,35.75 30.35,35.75 32.55,32.65 33.35,32.85 32.95,34.25 34.15,33.05 33.55,33.65 32.75,33.45
  pour Bottom (rank 2, no thermals): 42.55,36.55 34.85,36.55 34.35,35.75 34.25,35.65 33.65,35.65 32.55,36.35 25.25,36.35 25.25,34.55 31.15,34.55 31.15,30.45 33.45,30.45 34.55,31.35 39.05,34.55 42.55,34.55
  pour Top (rank 4, no thermals): 27.95,30.35 27.95,34.75 25.25,34.75 25.25,36.35 32.55,36.35 33.65,35.65 34.45,35.65 34.45,28.55 31.85,28.55 31.85,32.15 31.15,32.15 31.25,34.55 29.45,34.55 29.35,30.35
OB2  (via drill 0.4 pad 0.42)
  other vias: 26.35,32.65 25.55,32.65 27.15,32.65 25.95,33.35 26.75,33.35 26.35,34.05 30.05,32.65 30.45,33.35 30.05,34.05 29.75,29.65 30.45,29.25 29.05,29.25
  pour Bottom (no thermals): 42.55,34.25 38.85,34.25 35.25,31.55 33.55,30.25 31.05,30.25 31.05,34.55 25.65,34.55 25.65,33.65 25.25,33.45 25.25,30.35 28.65,30.35 28.65,27.05 33.95,27.05 42.55,32.05
  pour Top (rank 5, no thermals): 26.95,30.35 26.95,32.05 27.85,32.05 27.85,34.55 25.65,34.55 25.65,33.65 25.25,33.45 25.25,30.35
  pour Top (rank 3, no thermals): 29.55,34.55 29.45,30.25 28.45,30.25 28.45,28.55 31.05,28.55 31.15,34.55
RESET  (via drill 0.3)
  Top 0.152: J14.10 16.69,29.54 16.05,28.9 11.05,28.9 10.05,29.9 10.05,30.3 v10.15,30.4 | v9.25,33.6 8.75,34.1 8,34.1 | 8,34.1 | 5.85,40.55 v5.76,40.64 5.76,39.99 6.75,39 6.75,34.25 7.45,33.55 | R7.1 4.85,46.9 3.45,45.5 3.45,43.81 S2.P$1 | 8,34.1 7.98,34.08 7.45,33.55 | 7.45,33.55 7.2,33.3 U$1.52
  Bottom 0.152: v10.15,30.4 10.15,32.7 v9.25,33.6 | R7.1 6.95,46.65 8,45.6 8,42.89 v5.76,40.64
  other vias: 6.95,46.9
SRA
  Top 0.152: C30.2 R8.2 24.35,41.25 U$3.12
SRB
  Top 0.152: C31.2 R3.2 24.35,32.65 U$3.22
STEP  (via drill 0.3, 0.3 pad 0.42)
  Top 0.152: U$1.11 15.2,38.2 v15.34,38.06 | 35.03,39.35 U$3.42 35.05,39.35 34.62,38.92 34.62,38.62 33.75,37.75 33.11,37.75 v32.89,37.53
  Bottom 0.152: v15.34,38.06 15.45,38.06 15.7,37.82 17.38,37.82 17.87,37.33 18.14,37.33 18.96,36.51 23.9,36.51 24.7,37.31 32.65,37.31 32.88,37.53 v32.89,37.53
STLB  (via drill 0.3)
  Top 0.152: U$1.27 8.2,40.73 v8.34,40.59
  Bottom 0.152: v8.34,40.59 8.57,40.82 8.57,40.84 11.18,43.46 12.41,43.46 13.05,44.1 13.05,45.4 13.75,46.1 15.85,46.1 16.1,46.36 16.91,46.36 R5.1
  other vias: 17.35,46.8
STLR  (via drill 0.3)
  Top 0.152: U$1.26 8.7,41.05 v9.15,40.6
  Bottom 0.152: v9.15,40.6 9.15,40.8 11.45,43.1 15.15,43.1 15.65,43.6 15.65,45.4 16.25,46 17.95,46 R4.1
  other vias: 18.75,46.8
SWCLK
  Top 0.152: J14.4 12.88,29.53 12.65,29.3 11.25,29.3 10.75,29.8 10.75,30.77 9.84,31.68 9.84,31.71 9.75,31.8 9.75,32.4 U$1.57
SWDIO
  Top 0.152: J14.2 11.61,30.54 10.25,31.9 10.25,32.4 U$1.58
SWO
  Top 0.152: U$1.59 10.7,31.95 11.25,31.4 13.08,31.4 13.41,31.06 13.41,31.05 J14.6
TMC5VOUT
  Top 0.152: U$3.13 23.2,40.15 22.85,40.5 22.85,41.6 22.45,42 21.87,42 C4.1 20.74,42.81 19.95,43.6 19.95,45.1 20.35,45.5 20.35,49.1 20.65,49.4 21.95,49.4 25.15,52.6 25.15,53.77 S1.1
TMC_CSN  (via drill 0.3)
  Top 0.152: v16.54,40.16 13.99,40.16 U$1.15 | U$3.18 21.85,36.15 20.75,37.25 17.95,37.25 17.35,37.85 17.27,37.85 v16.54,38.58
  Bottom 0.152: v16.54,38.58 v16.54,40.16
TMC_EN
  Top 0.152: U$1.10 14.6,37.7 14.86,37.44 15.96,37.44 17.04,36.36 17.67,36.36 18.06,36.75 20.55,36.75 21.95,35.35 U$3.19
TMC_MISO
  Top 0.152: U$1.13 18.66,39.2 18.81,39.35 U$3.14
TMC_MOSI  (via drill 0.3)
  Top 0.152: v18.37,39.81 v18.36,39.81 17.3,40.87 16.16,40.87 15.99,40.7 U$1.16 | U$3.15 18.45,38.55 v18.41,38.59
  Bottom 0.152: v18.41,38.59 18.41,39.76 v18.37,39.81
TMC_SCK  (via drill 0.3)
  Top 0.152: U$1.14 14.58,39.7 14.73,39.56 17.2,39.56 v17.45,39.81 | v17.45,38.59 18.3,37.75 U$3.16
  Bottom 0.152: v17.45,38.59 v17.45,39.81
TMC_SG  (via drill 0.3, 0.3 pad 0.42)
  Top 0.152: U$1.9 14.6,37.2 14.71,37.08 15.35,37.08 v15.6,36.83 | v33.95,36.15 U$3.38
  Bottom 0.152: v15.6,36.83 16.46,36.83 16.93,36.36 18.1,36.36 18.67,35.79 24.2,35.79 25,36.59 32.98,36.59 33.21,36.37 33.73,36.37 v33.95,36.15
UP0RX  (via drill 0.3)
  Top 0.152: v7.45,40.1 7.45,40.7 7.25,40.9 7.25,41.4 U$1.29 | J12.P$2 6.66,6.84 7.5,6 8,6 8.5,6.5 8.5,11.49 v8.31,11.69
  Bottom 0.152: J8.P$2 7.3,10.65 v8.31,11.69 | v8.31,11.69 11.15,14.6 11.15,23.7 7.95,26.9 7.95,39.6 v7.45,40.1 | v8.31,11.69 | v8.31,11.69
UP0STLB  (via drill 0.3)
  Top 0.152: R10.1 9.5,19.25 10.25,20 10.25,23 8.5,24.75 4.5,24.75 2.75,26.5 2.75,30 v3,30.25 | U$1.36 5.7,39.2 v5.8,39.1
  Bottom 0.152: v3,30.25 3.25,30.25 4.25,31.25 4.25,34.25 4.32,34.32 4.32,35.05 4.3,35.07 4.3,38 5.01,38.71 5.51,38.71 5.8,39 v5.8,39.1
UP0STLR  (via drill 0.3)
  Top 0.152: U$1.38 v5.8,38.2 v5.81,38.19 | v3.33,29.44 3.33,29.33 3.11,29.11 3.11,26.65 4.65,25.11 8.65,25.11 10.61,23.15 10.61,18.29 R9.1
  Bottom 0.152: v5.81,38.19 5.39,38.19 4.66,37.46 4.66,35.21 4.67,35.2 4.67,31.17 3.65,30.15 3.65,29.76 v3.33,29.44
UP0TX  (via drill 0.3)
  Top 0.152: U$1.30 6.7,40.35 v6.55,40.2 | 7.65,10.5 v7.65,13.6 | 7.65,10.5 v7.65,6.9 | J12.P$5 7.5,10.65 7.65,10.5
  Bottom 0.152: v6.55,40.2 6.55,33.96 6.55,26.5 10.25,22.8 10.25,16.2 v7.65,13.6 | v7.65,6.9 4.5,6.9 J8.P$5
UP1RX  (via drill 0.3)
  Top 0.152: J13.P$2 27.41,6.84 28.25,6 28.5,6 29,6.5 29,10.51 v28.73,10.78 | v13.65,31.7 13.65,32 U$1.64
  Bottom 0.152: J10.P$2 28.61,10.65 v28.73,10.78 | v28.73,10.78 29.15,11.2 29.15,13.8 26.35,16.6 23.35,16.6 20.05,19.9 20.05,25.7 14.85,30.9 14.45,30.9 v13.65,31.7 | v28.73,10.78
UP1STLB  (via drill 0.3)
  Top 0.152: U$1.44 5.5,35.2 v5.8,35.5 | v4.04,27.87 4.04,27.74 3.82,27.52 3.82,26.94 4.94,25.82 8.94,25.82 11.32,23.44 11.32,19.69 12.35,18.65 13.25,18.65 R12.1
  Bottom 0.152: v5.8,35.5 5.7,35.5 5.38,35.19 5.38,30.88 4.36,29.85 4.36,28.19 v4.04,27.87
UP1STLR  (via drill 0.3)
  Top 0.152: R11.1 12.5,18 10.96,19.54 10.96,23.3 8.79,25.46 4.79,25.46 3.46,26.8 3.46,28.43 v3.69,28.66 | v5.8,37.3 5.8,36.4 5.6,36.2 U$1.42
  Bottom 0.152: v3.69,28.66 3.69,28.98 4.01,29.29 4.01,30 5.03,31.02 5.03,37.03 5.3,37.3 v5.8,37.3
UP1TX  (via drill 0.3)
  Top 0.152: 28.15,10.75 v28.15,13.3 | 28.15,10.75 28.15,7 v28.25,6.9 | J13.P$5 28.05,10.65 28.15,10.75 | U$1.63 12.6,32.55 12.6,32.87 11.87,33.6 v10.85,33.6
  Bottom 0.152: v28.15,13.3 25.85,15.6 21.75,15.6 19.45,17.9 19.45,19.96 19.63,20.14 19.63,22.94 19.15,23.42 19.15,24.5 11.45,32.2 11.45,33 v10.85,33.6 | v28.25,6.9 25.25,6.9 J10.P$5
USBDM  (via drill 0.3)
  Top 0.152: X1.D- 15.3,52.72 v13.79,51.21 | U$1.45 3.84,34.7 v3.74,34.81
  Bottom 0.152: v13.79,51.21 13.44,51.21 10.48,48.25 6.75,48.25 5.16,46.66 5.16,43.86 2.96,41.65 2.96,36.54 3.61,35.49 3.61,34.94 v3.74,34.81
USBDP  (via drill 0.3, 0.3 pad 0.42)
  Top 0.152: X1.D+ 14.65,52.92 v13.79,52.07 | v3.02,35.25 3.15,35.12 3.15,34.57 3.52,34.2 U$1.46
  Bottom 0.152: v13.79,52.07 10.33,48.61 6.6,48.61 4.8,46.81 4.8,44 2.6,41.8 2.6,36.08 v3.02,35.25
V+
  Top 0.2: C5.2 C6.1
  Top 0.305: U$3.30 31.55,31.25 31.55,36.55 31.57,36.53 32.94,36.53 33.29,36.18 33.29,35.88 33.68,35.49 34.11,35.49 34.54,35.06 34.54,34.95 34.95,34.55 U$3.36 37.45,34.55 C5.2
  Top 1.27: 33,24.7 C20.1
  Top 2.54: J2.P$1 25.01,21.54 26.65,19.9 30.35,19.9 32.55,22.1 32.55,24.25 33,24.7
  pour Top (no thermals): 34.75,49.45 32.95,51.35 31.15,51.35 31.15,22.65 33.05,22.65 34.85,24.55 34.85,28.45 31.85,28.45 31.85,45.55 34.75,45.55

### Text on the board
tPlace: mkstepper v0.2 | usb < - > tmc | GND | V+ | UP0 | UP1
bPlace: A1 | A2 | B1 | B2 | one at a time | UP0 | UP1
